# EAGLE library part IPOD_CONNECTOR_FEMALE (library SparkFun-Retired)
iPod Female Connector This is the connector found inside current iPods. Use this connector to attach to iPod accessories like Nike+iPods, etc. Schematic and footprint are not yet production proven. Spark Fun Electronics SKU : DEV-08035
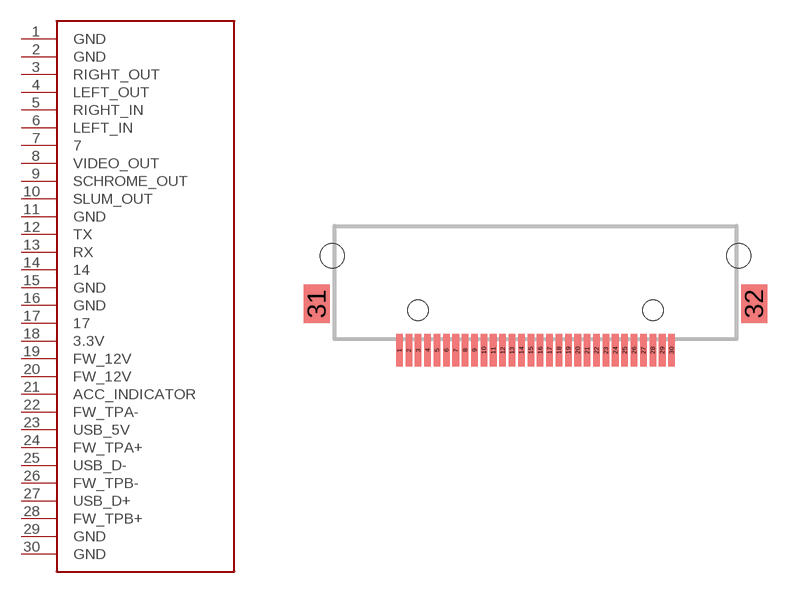
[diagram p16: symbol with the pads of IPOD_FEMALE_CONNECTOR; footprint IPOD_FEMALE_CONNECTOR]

Designator prefix -

## IPOD_CONNECTOR_FEMALE  [IPOD_FEMALE_CONNECTOR]
1  GND
2  GND
3  RIGHT_OUT
4  LEFT_OUT
5  RIGHT_IN
6  LEFT_IN
7  7
8  VIDEO_OUT
9  SCHROME_OUT
10  SLUM_OUT
11  GND
12  TX
13  RX
14  14
15  GND
16  GND
17  17
18  3.3V
19  FW_12V
20  FW_12V
21  ACC_INDICATOR
22  FW_TPA-
23  USB_5V
24  FW_TPA+
25  USB_D-
26  FW_TPB-
27  USB_D+
28  FW_TPB+
29  GND
30  GND

## Footprint IPOD_FEMALE_CONNECTOR (pad centres in mm)
smd 0.35 x 1.75: 1 -7.25,0; 2 -6.75,0; 3 -6.25,0; 4 -5.75,0; 5 -5.25,0; 6 -4.75,0; 7 -4.25,0; 8 -3.75,0; 9 -3.25,0; 10 -2.75,0; 11 -2.25,0; 12 -1.75,0; 13 -1.25,0; 14 -0.75,0; 15 -0.25,0; 16 0.25,0; 17 0.75,0; 18 1.25,0; 19 1.75,0; 20 2.25,0; 21 2.75,0; 22 3.25,0; 23 3.75,0; 24 4.25,0; 25 4.75,0; 26 5.25,0; 27 5.75,0; 28 6.25,0; 29 6.75,0; 30 7.25,0
smd 1.4 x 2.05: 31 -11.65,2.475; 32 11.65,2.475
hole 1.1 at 6.25,2.125
hole 1.1 at -6.25,2.125
hole 1.3 at 10.825,5.025
hole 1.3 at -10.825,5.025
